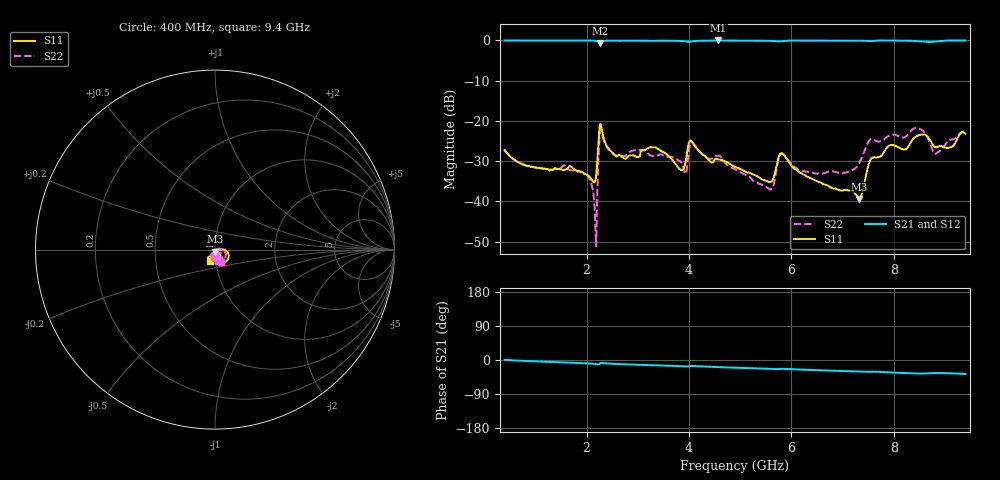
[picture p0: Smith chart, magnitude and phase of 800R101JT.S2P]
!  American Technical Ceramics  Date:  6/19/09
!  One Norden Lane
!  Huntington Station,  NY.  11746-2102
!  Tel:  (631) 622-4700  Fax:  (631) 622-4748
!  Part Number  800R101JT
!  Description: Ultra-low ESR, NPO  Mounting Orientation: Vertical
!  Application: High RF power Filters, Combiners, Matching networks,
!  Antenna, DC block, Bypass and Couplers
# GHZ S DB R 50
! Freq  |S11|  S11 Ph  |S21|  S21 Ph  |S12|  S12 Ph  |S22|  S22 Ph
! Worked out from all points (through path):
!   801 points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, 400 MHz to 9.4 GHz, reference 50 ohm
!   highest |S21| = 0.00 dB at 4.574 GHz (marker M1); lowest = -0.7 dB at 2.268 GHz (marker M2)
!   group delay of S21, straight-line fit = 11.3 ps
!   lowest |S11| = -39.4 dB at 7.33 GHz (marker M3), VSWR 1.02, Z = 50.1 - j1.07 ohm
!   |S11| at or under -10 dB: start of sweep to end of sweep
!   |S22| runs from -51.1 to -21.8 dB; largest |S21 - S12| = 0.0019
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0.4  -27.27 -88.4  -0.01 0.4  -0.02 0.5  -27.27 -89.1
1.908  -32.70 -79.2  -0.02 -8.2  -0.03 -8.2  -32.63 -112.5
2.076  -34.16 -65.9  -0.04 -9.3  -0.04 -9.3  -34.87 -119.6
2.166  -35.03 -31.0  -0.08 -10.3  -0.09 -10.3  -43.64 -113.7
2.2  -31.96 -5.5  -0.16 -11.0  -0.16 -11.0  -43.28 11.0
2.268  -20.78 -37.8  -0.68 -8.7  -0.69 -8.7  -22.38 -41.5
2.74  -29.32 -77.0  -0.06 -11.3  -0.06 -11.3  -28.72 -111.5
3.404  -27.02 -92.0  -0.07 -14.2  -0.08 -14.2  -28.48 -113.9
3.843  -32.19 -75.7  -0.12 -16.6  -0.12 -16.6  -30.19 -116.8
3.933  -30.35 -48.3  -0.22 -17.3  -0.22 -17.2  -33.22 -99.7
4.034  -24.86 -69.6  -0.31 -15.8  -0.31 -15.8  -25.60 -92.0
4.574  -29.59 -86.3  0.00 -18.8  0.00 -18.8  -28.64 -122.0
4.9  -31.43 -90.8  -0.04 -20.4  -0.04 -20.4  -31.99 -124.5
5.598  -35.17 -67.2  -0.10 -23.6  -0.10 -23.6  -37.06 -76.2
5.823  -28.11 -82.2  -0.18 -23.3  -0.18 -23.2  -28.11 -78.3
6.408  -34.38 -117.1  -0.01 -26.4  -0.01 -26.3  -32.84 -86.7
7.33  -39.38 -83.9  -0.04 -30.7  -0.04 -30.6  -30.47 -33.7
7.555  -29.48 -69.8  -0.14 -31.0  -0.14 -30.9  -24.51 -46.4
7.904  -26.19 -92.9  -0.01 -32.8  -0.01 -32.7  -23.70 -59.7
8.5  -23.51 -112.2  -0.21 -35.7  -0.20 -35.7  -21.94 -86.5
8.826  -26.59 -123.7  -0.26 -34.2  -0.26 -34.2  -28.09 -83.1
9.4  -23.17 -115.9  -0.01 -37.0  -0.01 -37.0  -22.44 -64.4
